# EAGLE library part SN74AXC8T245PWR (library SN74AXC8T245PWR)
8-Bit Dual-Supply Bus Transceiver Source: Datasheet
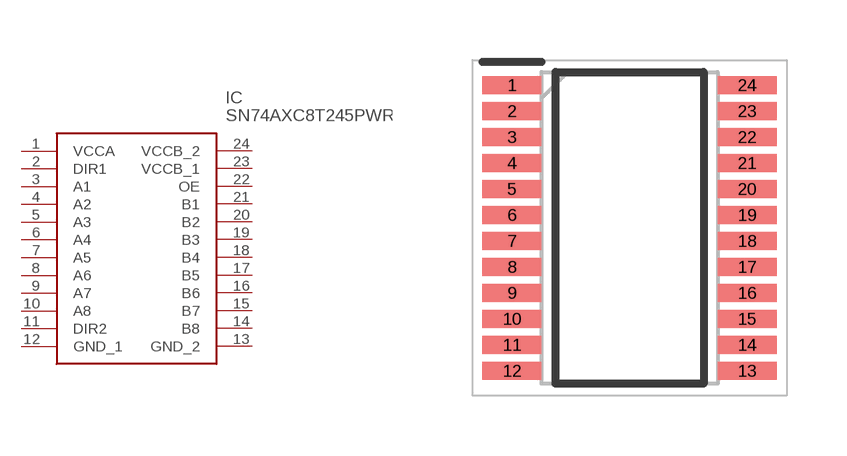
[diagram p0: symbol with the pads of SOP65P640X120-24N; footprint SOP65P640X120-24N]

Designator prefix IC

## SN74AXC8T245PWR (Description: 8-Bit Dual-Supply Bus Transceiver; Height: 1.2mm; Manufacturer_Name: Texas Instruments; Manufacturer_Part_Number: SN74AXC8T245PWR; Mouser_Part_Number: 595-SN74AXC8T245PWR; Mouser_Price-Stock: https://www.mouser.co.uk/ProductDetail/Texas-Instruments/SN74AXC8T245PWR?qs=r5DSvlrkXmJAK4f7nnPNow%3D%3D)  [SOP65P640X120-24N]
1  VCCA  pwr
2  DIR1  in
3  A1
4  A2
5  A3
6  A4
7  A5
8  A6
9  A7
10  A8
11  DIR2  in
12  GND_1  pwr
13  GND_2  pwr
14  B8
15  B7
16  B6
17  B5
18  B4
19  B3
20  B2
21  B1
22  OE  in
23  VCCB_1  pwr
24  VCCB_2  pwr

## Footprint SOP65P640X120-24N (pad centres in mm)
24-Pin TSSOP
smd 1.475 x 0.45: 1 -2.938,3.575; 2 -2.938,2.925; 3 -2.938,2.275; 4 -2.938,1.625; 5 -2.938,0.975; 6 -2.938,0.325; 7 -2.938,-0.325; 8 -2.938,-0.975; 9 -2.938,-1.625; 10 -2.938,-2.275; 11 -2.938,-2.925; 12 -2.938,-3.575; 13 2.938,-3.575; 14 2.938,-2.925; 15 2.938,-2.275; 16 2.938,-1.625; 17 2.938,-0.975; 18 2.938,-0.325; 19 2.938,0.325; 20 2.938,0.975; 21 2.938,1.625; 22 2.938,2.275; 23 2.938,2.925; 24 2.938,3.575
